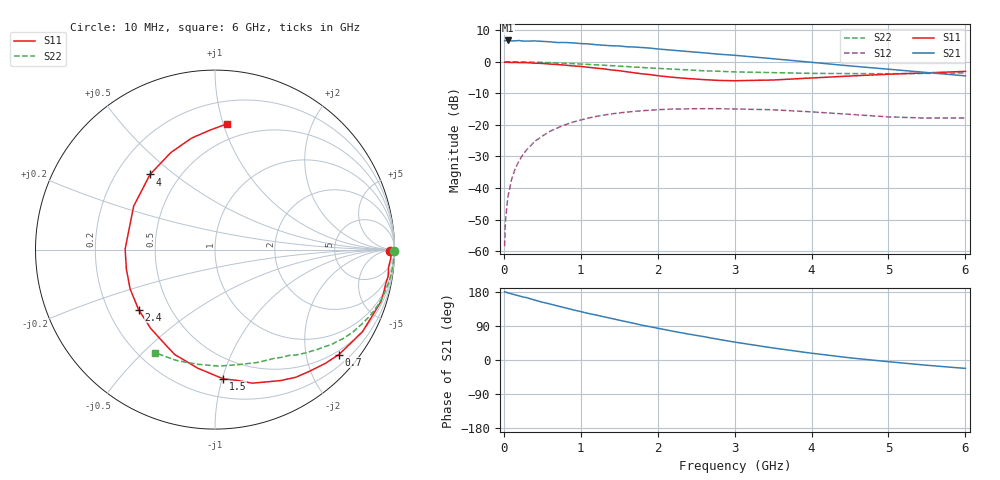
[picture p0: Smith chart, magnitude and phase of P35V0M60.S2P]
! SIEMENS Small Signal Semiconductors
! BFP181
! Si NPN RF Bipolar Junction Transistor in SOT143
! VCE = 5 V  IC = 0.6 mA
! Common Emitter S-Parameters:  March  1996
# GHz  S  MA  R  50
!  f  S11  S21  S12  S22
! GHz  MAG  ANG  MAG  ANG  MAG  ANG  MAG  ANG
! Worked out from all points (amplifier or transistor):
!   36 points, 10 MHz to 6 GHz, reference 50 ohm
!   highest |S21| = 6.7 dB at 50 MHz (marker M1)
!   |S21| within 3 dB of that: start of sweep to 2.15 GHz
!   unconditionally stable (mu >= 1): 3.698 GHz to end of sweep
!   at 250 MHz: K = 0.08, MSG = 17.9 dB, |S12| = -29.3 dB
!   at 1.4 GHz: K = 0.43, MSG = 10.8 dB, |S12| = -16.5 dB
!   at 6 GHz: K = 1.40, MAG = 2.9 dB, |S12| = -17.8 dB
!   S11 on the Smith chart (normalised r, x): 10 MHz: 72, -32; 700 MHz: 0.41, -2.67; 1.5 GHz: 0.34, -1.01; 2.4 GHz: 0.33, -0.31; 4 GHz: 0.34, +0.41; 6 GHz: 0.37, +1.03
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0.01  0.9771 -0.6  2.155 179.7  0.0012 76.1  0.9996 -0.3
0.02  0.9811 -1.2  2.152 179.6  0.0029 94.4  0.9987 -0.6
0.05  0.9811 -2.7  2.174 177.2  0.0069 90.9  0.9977 -1.5
0.1  0.9722 -5.8  2.14 174.6  0.0136 84.2  0.9974 -2.8
0.15  0.9761 -8.7  2.146 171.8  0.0207 83.0  0.9957 -4.2
0.2  0.97 -11.5  2.168 169.1  0.0271 81.7  0.9948 -5.6
0.25  0.9699 -14.5  2.126 166.3  0.0342 80.1  0.9921 -7.0
0.3  0.9688 -17.4  2.123 164.4  0.0407 77.6  0.9903 -8.3
0.4  0.9496 -23.3  2.137 158.1  0.0544 73.8  0.9843 -11.1
0.7  0.9047 -40.3  2.016 142.6  0.0901 61.9  0.9581 -19.0
0.9  0.8593 -51.9  1.99 132.4  0.1109 54.2  0.9336 -24.0
1.1  0.8166 -63.3  1.918 122.8  0.1283 47.3  0.907 -28.6
1.5  0.7214 -86.4  1.778 105.0  0.1546 34.8  0.8514 -36.8
1.9  0.6265 -110.9  1.645 87.9  0.1707 23.8  0.7972 -44.2
2.2  0.5667 -129.2  1.521 75.8  0.178 16.9  0.7636 -49.0
2.4  0.5414 -141.8  1.449 68.5  0.18 12.3  0.7418 -52.3
3  0.5006 179.7  1.266 47.3  0.1788 1.0  0.6902 -61.3
3.5  0.5138 151.9  1.116 31.7  0.1736 -6.1  0.6728 -69.0
4  0.5535 130.8  0.98 17.9  0.1606 -11.4  0.6548 -78.1
4.5  0.5943 114.4  0.859 5.7  0.1469 -14.7  0.6494 -88.3
5.5  0.667 92.2  0.675 -13.9  0.1281 -11.1  0.654 -109.3
6  0.7041 84.5  0.598 -22.2  0.1288 -7.5  0.6647 -120.3
